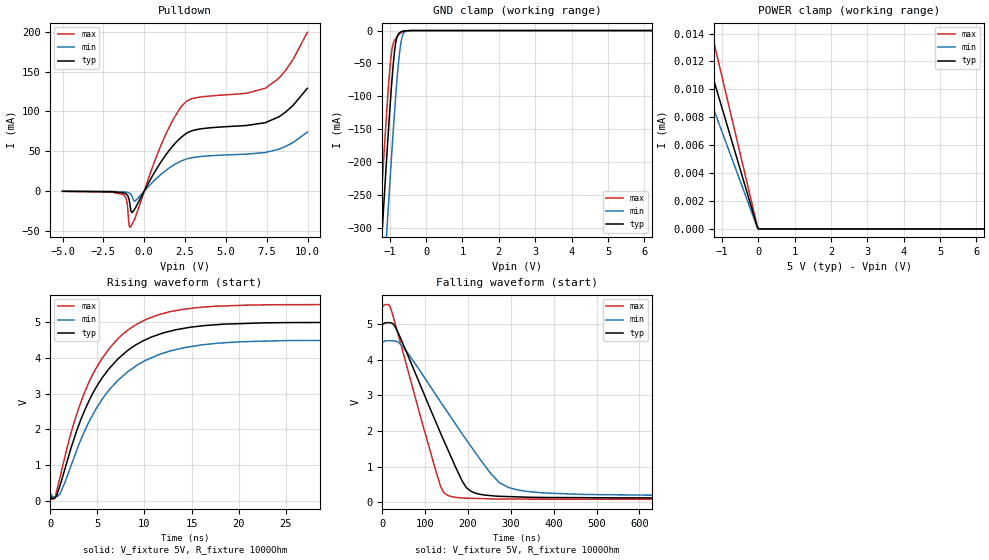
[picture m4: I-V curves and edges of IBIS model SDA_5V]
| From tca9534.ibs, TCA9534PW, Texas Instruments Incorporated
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[Model]   SDA_5V
Model_type   I/O_open_drain
Polarity   Non-Inverting
Enable   Active-Low
Vinl = .8
Vinh = 2
Vmeas = 2.5
Vref = 5
Cref = 15pF
Rref = 1000
|   typ   min   max
|   (nom PVT)   (slow PVT)   (fast PVT)
C_comp   1.467p   1.400p   1.599p
|C_comp (ON state)   1.550p   1.468p   1.684p
|C_comp (OFF state)   1.467p   1.400p   1.599p
| Where   nom PVT is  Nominal Process, 5.0V, 27C
|   Fast PVT is Strong Process, 5.5V, -40C
|   Slow PVT is Weak Process, 4.5V, 125C
[Voltage Range]   5   4.5   5.5
[Temperature Range]   27   125   -40
[Pullup Reference]   5   4.5   5.5
[Pulldown Reference]   -0   -0   -0
[Power Clamp Reference]   5   4.5   5.5
[GND Clamp Reference]   -0   -0   -0
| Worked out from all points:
|   slope of the pulldown table from 0 to 0.75 V, typ, clamps not added: 27.1 ohm
|   GND clamp passes 1 mA (typ) near -0.63 V on its own axis
|   falling waveform, V_fixture 5V, R_fixture 1000Ohm: 20-80 % time 104ns typ, 147ns min, 74.6ns max; typ from 5 V to 0.119 V
|   rising waveform, V_fixture 5V, R_fixture 1000Ohm: 20-80 % time 5.62ns typ, 6.04ns min, 5.27ns max; typ from 0.119 V to 5 V
[Pulldown]
|   Voltage   I(typ)   I(min)   I(max)
-5V       -178uA     -88.8uA    -261.6uA
-1.25V    -2.203mA   -868uA     -4.427mA
-1.055V   -4.48mA    -1.402mA   -13.93mA
-935mV    -9.719mA   -2.153mA   -41.05mA
-860mV    -18.62mA   -3.09mA    -45.01mA
-755mV    -26.81mA   -6.104mA   -41.83mA
-545mV    -21.1mA    -12.15mA   -32.85mA
1.06V     37.74mA    21.65mA    59.27mA
2.32V     68.53mA    38.32mA    107.2mA
7.42V     86.03mA    48.54mA    129.3mA
8.65V     99.19mA    56.13mA    151.5mA
9.985V    129.1mA    74.03mA    199.3mA
[GND Clamp]
|   Voltage   I(typ)   I(min)   I(max)
-5V       -4.031A    -4.136A    -3.967A
-1.43V    -515.4mA   -631.4mA   -442.9mA
-1.25V    -346.1mA   -462.2mA   -273.4mA
-1.145V   -249.9mA   -365.4mA   -178.2mA
-1.1V     -209.7mA   -324.6mA   -139.1mA
-1.055V   -170.5mA   -284.2mA   -102mA
-965mV    -96.56mA   -205.6mA   -40.65mA
-860mV    -29.03mA   -119.8mA   -14.61mA
-740mV    -4.086mA   -39.8mA    -6.122mA
-665mV    -1.534mA   -11.59mA   -2.683mA
-410mV    -15.77uA   -33.89uA   -17.88uA
9.985V    0A         0A         0A
[POWER Clamp]
|   Voltage   I(typ)   I(min)   I(max)
-5V       2.642mA    2.712mA    3.638mA
-2.015V   20.5uA     14.31uA    205.4uA
-1.775V   15.55uA    12.51uA    22.26uA
-1.25V    10.94uA    8.79uA     13.75uA
-20mV     121.3nA    88.28nA    169.5nA
10mV      0A         0A         56.49nA
25mV      0A         0A         0A
9.985V    0A         0A         0A
[Ramp]
R_load = 1000
|   typ   min   max
dV/dt_r   2.92862/5.61255e-09   2.5886/6.05178e-09   3.25109/5.25338e-09
dV/dt_f   2.9285/1.03936e-07   2.58764/1.47313e-07   3.25108/7.45524e-08
[Falling Waveform]
V_fixture = 5V
V_fixture_min = 4.5V
V_fixture_max = 5.5V
R_fixture = 1000Ohm
C_fixture = 0F
|   Time   V(typ)   V(min)   V(max)
0s        5V         4.5V       5.5V
19.32ns   5.03V      4.526V     5.439V
45.93ns   4.5V       4.387V     4.303V
123.8ns   2.278V     3.03V      919.8mV
136.1ns   1.931V     2.808V     439.6mV
151.6ns   1.507V     2.53V      199.1mV
206.4ns   308.9mV    1.57V      110.6mV
274.3ns   165.6mV    539.4mV    90.88mV
314.3ns   150.7mV    347.9mV    88.31mV
999.9ns   119.2mV    187.3mV    81.54mV
[Rising Waveform]
V_fixture = 5V
V_fixture_min = 4.5V
V_fixture_max = 5.5V
R_fixture = 1000Ohm
C_fixture = 0F
|   Time   V(typ)   V(min)   V(max)
0s        119mV      185.7mV    81.52mV
455ps     74.27mV    104.1mV    66.61mV
1.039ns   429.6mV    196.7mV    664.5mV
2.374ns   1.615V     1.103V     2.057V
3.93ns    2.696V     2.113V     3.219V
5.431ns   3.414V     2.813V     3.961V
7.312ns   4.003V     3.406V     4.575V
12.78ns   4.756V     4.201V     5.301V
21.22ns   4.973V     4.463V     5.485V
999.9ns   5V         4.5V       5.5V
